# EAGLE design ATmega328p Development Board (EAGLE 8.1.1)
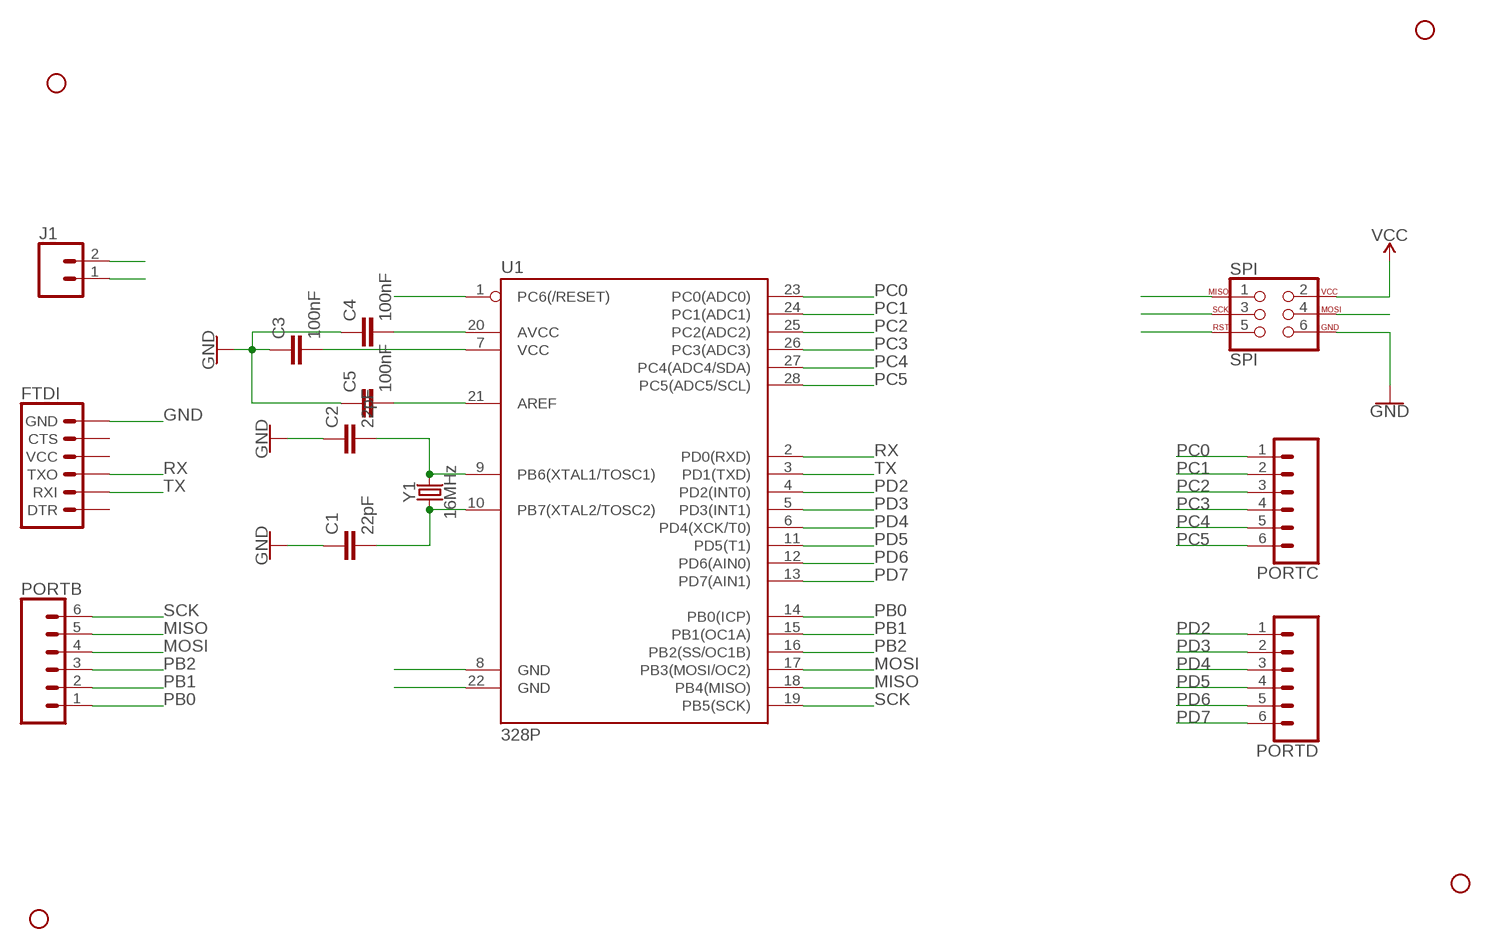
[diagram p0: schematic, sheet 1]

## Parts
C1  22pF  1.0UF-0805-25V-10%  [0805]
C2  22pF  1.0UF-0805-25V-10%  [0805]
C3  100nF  1.0UF-0805-25V-10%  [0805]
C4  100nF  1.0UF-0805-25V-10%  [0805]
C5  100nF  1.0UF-0805-25V-10%  [0805]
FTDI  6_PIN_SERIAL_TARGET  [1X06]
H1  STAND-OFF  [STAND-OFF]
H2  STAND-OFF  [STAND-OFF]
H3  STAND-OFF  [STAND-OFF]
H4  STAND-OFF  [STAND-OFF]
J1  CONN_02  [1X02]
PORTB  CONN_06SILK_FEMALE_PTH  [1X06]
PORTC  CONN_06SILK_FEMALE_PTH  [1X06]
PORTD  CONN_06SILK_FEMALE_PTH  [1X06]
SPI  SPI  AVR_SPI_PROG_3X2NS  [2X3-NS]
U1  328P  ATMEGA328P_PDIP  [DIP28]
Y1  16MHz  CRYSTAL-16MHZPTH-HC49US  [HC49US]

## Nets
AREF: C5.2 U1.21(AREF)
GND: C1.1 C2.1 C3.1 C4.1 C5.1 FTDI.6(GND) J1.1 SPI.6 U1.8(GND) U1.22(GND)
MISO: PORTB.5 SPI.1 U1.18(PB4(MISO))
MOSI: PORTB.4 SPI.4 U1.17(PB3(MOSI/OC2))
N$1: C1.2 U1.10(PB7(XTAL2/TOSC2)) Y1.1
N$2: C2.2 U1.9(PB6(XTAL1/TOSC1)) Y1.2
PB0: PORTB.1 U1.14(PB0(ICP))
PB1: PORTB.2 U1.15(PB1(OC1A))
PB2: PORTB.3 U1.16(PB2(SS/OC1B))
PC0: PORTC.1 U1.23(PC0(ADC0))
PC1: PORTC.2 U1.24(PC1(ADC1))
PC2: PORTC.3 U1.25(PC2(ADC2))
PC3: PORTC.4 U1.26(PC3(ADC3))
PC4: PORTC.5 U1.27(PC4(ADC4/SDA))
PC5: PORTC.6 U1.28(PC5(ADC5/SCL))
PD2: PORTD.1 U1.4(PD2(INT0))
PD3: PORTD.2 U1.5(PD3(INT1))
PD4: PORTD.3 U1.6(PD4(XCK/T0))
PD5: PORTD.4 U1.11(PD5(T1))
PD6: PORTD.5 U1.12(PD6(AIN0))
PD7: PORTD.6 U1.13(PD7(AIN1))
RST: SPI.5 U1.1(PC6(/RESET))
RX: FTDI.3(TXO) U1.2(PD0(RXD))
SCK: PORTB.6 SPI.3 U1.19(PB5(SCK))
TX: FTDI.2(RXI) U1.3(PD1(TXD))
VCC: C3.2 C4.2 J1.2 SPI.2 U1.7(VCC) U1.20(AVCC)
Unconnected: FTDI.1(DTR) FTDI.4(VCC) FTDI.5(CTS)

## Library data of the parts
C1-C5 = SparkFun-Capacitors:1.0UF: 1µF ceramic capacitors; PROD_ID: CAP-08064; VALUE: 1.0uF
FTDI = SparkFun-Connectors:6_PIN_SERIAL_TARGET: 6-pin header connection for use with the "FTDI BASIC" pinout - TARGET SIDE. Also known as "Arduino Serial Program Header". It is used to mate with our FTDI Basic serial programmers using the Arduino IDE. Note, this device has "TARGET" in the name. It is intended to be used on a design that contains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
H1-H4 = SparkFun-Hardware:STAND-OFF: Stand Off
J1 = SparkFun-Connectors:CONN_02: Multi connection point. Often used as Generic Header-pin footprint for 0.1 inch spaced/style header connections
PORTB PORTC PORTD = SparkFun-Connectors:CONN_06: Multi connection point. Often used as Generic Header-pin footprint for 0.1 inch spaced/style header connections On any of the 0.1 inch spaced packages, you can populate with these: Break Away Headers - Straight (PRT-00116) Break Away Male Headers - Right Angle (PRT-00553) Female Headers (PRT-00115)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; PROD_ID: CONN-08437
SPI = SparkFun-Connectors:AVR_SPI_PROG_3X2: AVR ISP 6 Pin This is the reduced ISP connector for AVR programming. Common on Arduino. This footprint will take up less PCB space and can be used with a 10-pin to 6-pin adapter such as SKU: BOB-08508 **Special note about "TEST_POINT" package. The stop mask is on the top side, so if you want your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
U1 = SparkFun-IC-Microcontroller:ATMEGA328P_PDIP: Atmel 328P Through hole ATMEGA328P uC used in the Arduino 32kb flash, 1k EEPROM, 2k SRAM Datasheet SparkFun Products Storefront component: AVR 28 Pin 20MHz 32K 6A/D - ATMega328P (COM-09061) SparkFun Simon Says - Through-Hole Soldering Kit (KIT-10547) SparkFun Learn to Solder - Simon Says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; PROD_ID: IC-09136
Y1 = SparkFun-Clocks:CRYSTAL-16MHZ: 16MHz Crystal; PROD_ID: XTAL-08181; SF_ID: COM-00536

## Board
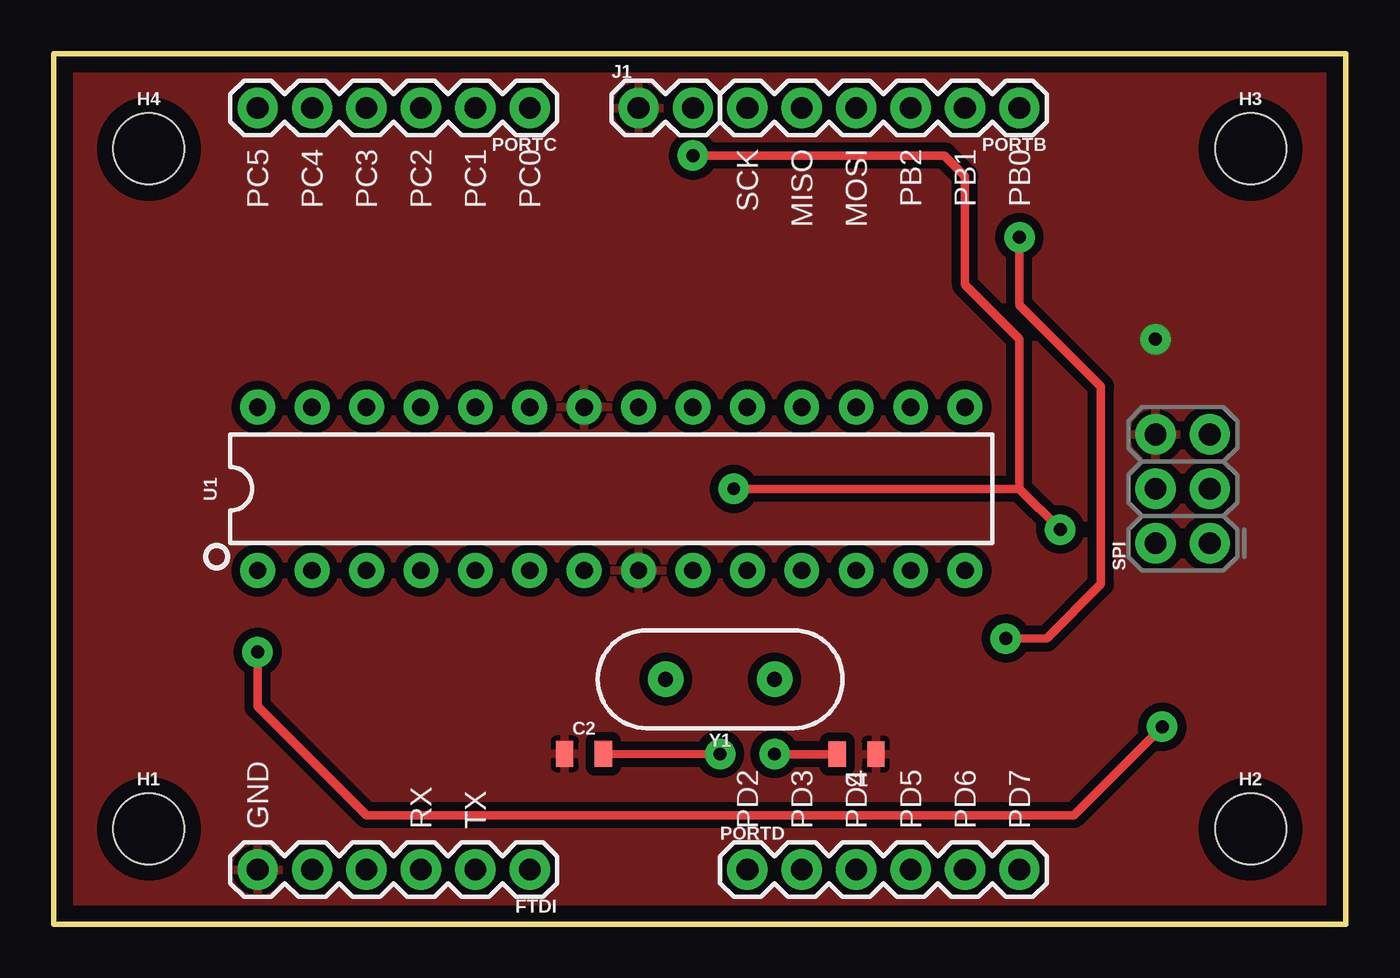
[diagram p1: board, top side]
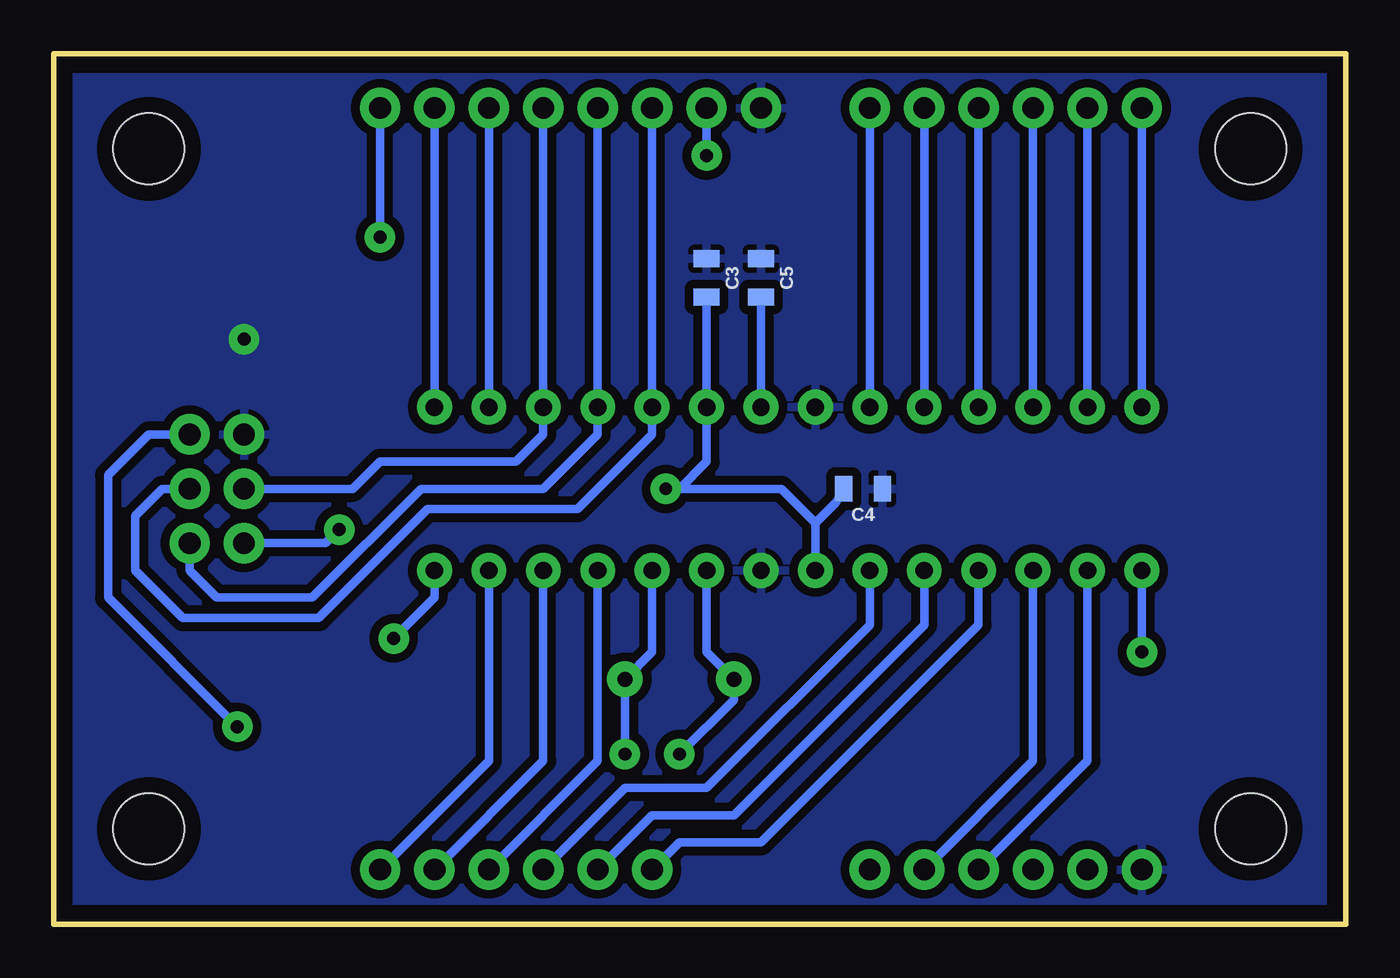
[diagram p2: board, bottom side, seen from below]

Size 60.33 x 40.64 mm. Coordinates in mm from the lower left corner, seen from the top.
Outline: 0,0 60.33,0 60.33,40.64 0,40.64 0,0
Copper layers (1*16): Top 0.035mm / dielectric 1.5mm / Bottom 0.035mm
Design rules "default *": minimum track width 10mil, minimum drill 24mil, track to track 8mil, track to pad 8mil, pad to pad 8mil, via to via 8mil, smd to smd 8mil, copper to edge 30mil, drill to drill 8mil, minimum pad ring 10mil, minimum via ring 8mil, stop-mask expansion 4mil, vias tented up to drill 0mil, thermal gap 10mil

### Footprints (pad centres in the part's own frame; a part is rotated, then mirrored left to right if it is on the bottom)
0805 = smd 0.8 x 1.2: 1 -0.9,0; 2 0.9,0
1X06 = drill 1.016 pad 1.88: 1 0,0; 2 2.54,0; 3 5.08,0; 4 7.62,0; 5 10.16,0; 6 12.7,0
STAND-OFF = hole 3.302: 0,0
1X02 = drill 1.016 pad 1.88: 1 0,0; 2 2.54,0
2X3-NS = drill 1.016 pad 1.88: 1 -2.54,-1.27; 2 -2.54,1.27; 3 0,-1.27; 4 0,1.27; 5 2.54,-1.27; 6 2.54,1.27
DIP28 = drill 0.813 pad 1.626: 1 -16.51,-3.81; 2 -13.97,-3.81; 3 -11.43,-3.81; 4 -8.89,-3.81; 5 -6.35,-3.81; 6 -3.81,-3.81; 7 -1.27,-3.81; 8 1.27,-3.81; 9 3.81,-3.81; 10 6.35,-3.81; 11 8.89,-3.81; 12 11.43,-3.81; 13 13.97,-3.81; 14 16.51,-3.81; 15 16.51,3.81; 16 13.97,3.81; 17 11.43,3.81; 18 8.89,3.81; 19 6.35,3.81; 20 3.81,3.81; 21 1.27,3.81; 22 -1.27,3.81; 23 -3.81,3.81; 24 -6.35,3.81; 25 -8.89,3.81; 26 -11.43,3.81; 27 -13.97,3.81; 28 -16.51,3.81
HC49US = drill 0.7 pad 1.651: 1 -2.54,0; 2 2.54,0

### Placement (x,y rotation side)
C1  37.48,7.93 180 top
C2  24.76,7.95 0 top
C3  29.84,30.16 270 bottom
C4  22.54,20.32 180 bottom
C5  27.3,30.16 270 bottom
FTDI  22.23,2.54 180 top
H1  4.45,4.45 0 top
H2  55.88,4.45 0 top
H3  55.88,36.2 0 top
H4  4.45,36.2 0 top
J1  27.3,38.1 0 top
PORTB  45.09,38.1 180 top
PORTC  22.23,38.1 180 top
PORTD  32.38,2.54 0 top
SPI  52.7,20.32 90 top
U1  26.04,20.32 0 top
Y1  31.11,11.43 180 top

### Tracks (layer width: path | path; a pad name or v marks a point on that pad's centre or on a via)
AREF
  Bottom 0.406: U1.21 C5.2
GND  (via drill 0.6 pad 1.42)
  other vias: 51.44,27.3
  pour Top (isolate 0.406): 0,40.64 60.33,40.64 60.33,0 0,0
  pour Bottom (isolate 0.406): 0,40.64 60.33,40.64 60.33,0 0,0
MISO
  Bottom 0.406: PORTB.5 U1.18 34.92,22.86 37.47,20.32 43.18,20.32 48.26,15.24 52.7,15.24 53.98,16.51 SPI.1
MOSI
  Bottom 0.406: PORTB.4 U1.17 37.47,22.86 38.73,21.59 45.09,21.59 46.35,20.32 SPI.4
N$1  (via drill 0.6 pad 1.42)
  Top 0.406: C1.2 33.97,7.93 v33.66,7.94
  Bottom 0.406: U1.10 32.38,12.7 Y1.1 v33.66,7.94
N$2  (via drill 0.6 pad 1.42)
  Top 0.406: C2.2 31.1,7.92 v31.11,7.94
  Bottom 0.406: U1.9 29.84,12.7 Y1.2 28.57,10.48 v31.11,7.94
N$7
  pour Bottom (isolate 0.406): 0,0 60.33,0 60.33,40.64 0,40.64
N$8
  pour Top (isolate 0.406): 0,0 60.33,0 60.33,40.64 0,40.64
PB0  (via drill 0.6 pad 1.42)
  Top 0.406: v44.45,13.34 46.35,13.34 48.9,15.88 48.9,25.08 45.09,28.89 v45.09,32.07
  Bottom 0.406: U1.14 42.55,15.24 v44.45,13.34 | v45.09,32.07 PORTB.1
PB1
  Bottom 0.406: PORTB.2 U1.15
PB2
  Bottom 0.406: PORTB.3 U1.16
PC0
  Bottom 0.406: PORTC.1 U1.23
PC1
  Bottom 0.406: U1.24 PORTC.2
PC2
  Bottom 0.406: PORTC.3 U1.25
PC3
  Bottom 0.406: U1.26 PORTC.4
PC4
  Bottom 0.406: PORTC.5 U1.27
PC5
  Bottom 0.406: U1.28 PORTC.6
PD2
  Bottom 0.406: PORTD.1 31.11,3.81 27.3,3.81 17.14,13.97 U1.4
PD3
  Bottom 0.406: PORTD.2 32.38,5.08 28.57,5.08 19.68,13.97 U1.5
PD4
  Bottom 0.406: PORTD.3 33.66,6.35 29.84,6.35 22.23,13.97 U1.6
PD5
  Bottom 0.406: PORTD.4 34.92,7.62 U1.11
PD6
  Bottom 0.406: PORTD.5 37.47,7.62 U1.12
PD7
  Bottom 0.406: PORTD.6 40.01,7.62 U1.13
RST  (via drill 0.6 pad 1.42)
  Top 0.406: v51.75,9.21 47.62,5.08 14.61,5.08 9.53,10.16 v9.53,12.7
  Bottom 0.406: SPI.5 55.88,22.86 57.78,20.95 57.78,15.24 v51.75,9.21 | 9.53,15.36 U1.1 v9.53,12.7 9.49,12.74
RX
  Bottom 0.406: FTDI.3 12.06,7.62 U1.2
SCK
  Bottom 0.406: PORTB.6 U1.19 32.38,22.86 35.88,19.37 42.86,19.37 47.94,14.29 54.29,14.29 56.52,16.51 56.52,19.05 55.24,20.32 SPI.3
TX
  Bottom 0.406: FTDI.2 14.61,7.62 U1.3
VCC  (via drill 0.6 pad 1.42)
  Top 0.406: 45.09,20.32 v31.75,20.32 | 45.09,20.32 v46.99,18.41 | 45.09,20.32 45.09,27.3 42.55,29.84 42.55,34.92 41.59,35.88 v29.84,35.88
  Bottom 0.406: 24.77,18.73 26.35,20.32 v31.75,20.32 31.11,20.32 29.84,21.59 U1.20 C3.2 | 24.77,18.73 U1.7 24.82,16.46 | SPI.2 47.62,17.78 v46.99,18.41 | J1.2 v29.84,35.88 | C4.2 23.81,19.68 24.77,18.73

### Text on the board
tPlace: PC5 | PC4 | PC3 | PC2 | PC1 | PC0 | SCK | MISO | MOSI | PB2 | PB1 | PB0 | GND | RX | TX | PD2 | PD3 | PD4 | PD5 | PD6 | PD7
